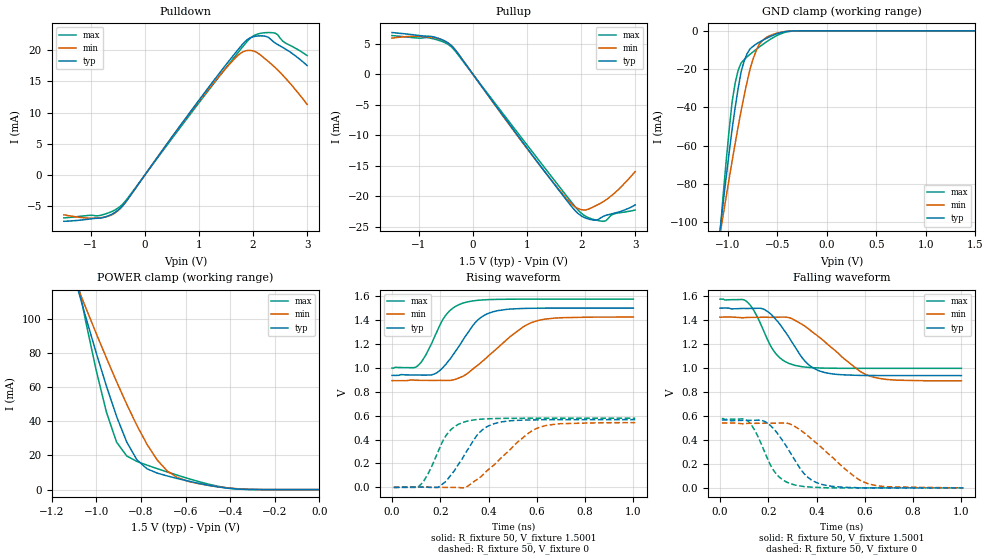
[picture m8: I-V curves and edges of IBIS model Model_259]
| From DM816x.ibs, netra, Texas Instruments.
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| Model based on original model for BSHTLTCSCDDVGPBFZ
|   Sub model FAST_5MA_5PER_P_1P5
[model]   Model_259
|[Description]  1.5V-3-STATE-X-FAST, 5MA, +-5%
|[Input Load]
|[Output Drive] FAST, 5MA
|Voltage   1.5V
|Mode   3-STATE
Model_type   3-state
Polarity   Non-Inverting
Enable   Active-Low
Cref =  15.0000pF
Rref =  100.0000M
Vref =  0V
Vmeas =  0.75005
C_comp   1.5249p   1.4275p   1.6205p
[Model Spec]
[Temperature Range]   25   125   -40
[Voltage Range]   1.5   1.425   1.575
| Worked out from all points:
|   slope of the pulldown table from 0 to 0.225 V, typ, clamps not added: 81.7 ohm
|   slope of the pullup table from 0 to 0.225 V, typ, clamps not added: 81.7 ohm
|   GND clamp passes 1 mA (typ) near -0.47 V on its own axis
|   POWER clamp passes 1 mA (typ) near -0.42 V on its own axis
|   rising waveform, R_fixture 50, V_fixture 1.5001: 20-80 % time 118ps typ, 187ps min, 89ps max; typ from 0.937 V to 1.5 V
|   rising waveform, R_fixture 50, V_fixture 0: 20-80 % time 112ps typ, 175ps min, 85.1ps max; typ from 0 V to 0.566 V
|   falling waveform, R_fixture 50, V_fixture 1.5001: 20-80 % time 117ps typ, 191ps min, 88.4ps max; typ from 1.5 V to 0.937 V
|   falling waveform, R_fixture 50, V_fixture 0: 20-80 % time 112ps typ, 184ps min, 84.9ps max; typ from 0.566 V to 0 V
[POWER_clamp]
-1.5V     321.7mA    260.6mA    415.9mA
-1.076V   114.2mA    115.8mA    116.9mA
-1.061V   107.2mA    110.9mA    107.1mA
-954.6mV  60.59mA    77.06mA    45.35mA
-909.2mV  42.85mA    63.21mA    27.81mA
-863.7mV  27.9mA     49.99mA    19.69mA
-818.2mV  17.49mA    37.63mA    16.52mA
-772.8mV  12.19mA    26.53mA    14.33mA
-681.9mV  7.985mA    10.89mA    10.33mA
-590.9mV  5.094mA    4.955mA    6.6mA
-363.7mV  298.5uA    465.2uA    297.6uA
0V        1.518nA    24.08nA    367.8pA
[Pulldown]
-1.5V     -7.45mA    -6.4mA     -6.9mA
-863.7mV  -6.95mA    -6.903mA   -6.565mA
-500mV    -5.682mA   -5.758mA   -5.339mA
-318.2mV  -3.897mA   -3.924mA   -3.728mA
1.046V    12.53mA    12.35mA    12.1mA
1.591V    18.69mA    18.02mA    18.2mA
1.818V    21.09mA    19.78mA    20.66mA
1.955V    22.02mA    19.97mA    21.99mA
2.091V    22.3mA     19.54mA    22.62mA
2.273V    22.11mA    18.26mA    22.84mA
2.364V    21.46mA    17.58mA    22.81mA
3V        17.55mA    11.32mA    19.14mA
[Pullup]
-1.5V     6.87mA     5.96mA     6.38mA
-818.2mV  6.271mA    6.141mA    6.005mA
-590.9mV  5.763mA    5.741mA    5.469mA
-409.1mV  4.8mA      4.791mA    4.587mA
1.227V    -14.81mA   -14.84mA   -14.21mA
1.727V    -20.63mA   -20.37mA   -19.92mA
1.909V    -22.57mA   -21.88mA   -21.95mA
2.046V    -23.45mA   -22.28mA   -23.09mA
2.227V    -23.93mA   -21.76mA   -23.82mA
2.409V    -23.32mA   -20.9mA    -24.13mA
2.591V    -22.85mA   -19.7mA    -22.97mA
3V        -21.43mA   -15.95mA   -22.28mA
[GND_clamp]
-1.5V     -310.1mA   -250.5mA   -402.5mA
-1.076V   -103.6mA   -106.2mA   -105.2mA
-1.046V   -89.81mA   -96.36mA   -86.02mA
-954.6mV  -51.22mA   -67.87mA   -36.88mA
-924.3mV  -40.08mA   -58.86mA   -27.29mA
-863.7mV  -21.24mA   -41.56mA   -16.73mA
-833.4mV  -15.8mA    -33.75mA   -15.03mA
-772.8mV  -9.345mA   -19.75mA   -12.19mA
-712.2mV  -6.928mA   -10.35mA   -9.704mA
-621.3mV  -4.261mA   -3.896mA   -6.225mA
-409.1mV  -337.1uA   -289.1uA   -618.9uA
1.5V      1.518nA    257.2nA    299pA
[Ramp]
dV/dt_f   0.45084/0.17883415n   0.425896/0.27079683n   0.4624/0.14098927n
dV/dt_r 0.45449408/0.17056745n 0.43634864/0.25170346n 0.46290125/0.13634761n
R_load = 50
[Rising Waveform]
R_fixture = 50
V_fixture = 1.5001
V_fixture_min = 1.425
V_fixture_max = 1.575
0s        937.3mV    893.3mV    997.8mV
105.5ps   940.3mV    896mV      1.015V
140.9ps   939.6mV    895.5mV    1.11V
190.7ps   965.5mV    895.3mV    1.322V
236.6ps   1.063V     894.9mV    1.472V
297.2ps   1.242V     932.8mV    1.544V
345.4ps   1.379V     1.007V     1.563V
389ps     1.446V     1.08V      1.57V
580.2ps   1.499V     1.38V      1.575V
1ns       1.5V       1.425V     1.575V
[Rising Waveform]
R_fixture = 50
V_fixture = 0
V_fixture_min = 0
V_fixture_max = 0
7.64ps    0V         0V         0V
113ps     3.206mV    2.933mV    11.95mV
147.8ps   2.243mV    2.369mV    106.8mV
189.5ps   0V         0V         291mV
238ps     87.51mV    0V         469.6mV
308.9ps   300.8mV    4.48mV     552.9mV
357.8ps   448.4mV    72.85mV    568.7mV
407.3ps   521mV      162.2mV    574.8mV
604.8ps   565.2mV    497.7mV    578.4mV
1.008ns   566.5mV    541.4mV    578.6mV
[Falling Waveform]
R_fixture = 50
V_fixture = 1.5001
V_fixture_min = 1.425
V_fixture_max = 1.575
0s        1.5V       1.424V     1.575V
110.7ps   1.496V     1.421V     1.554V
144.1ps   1.497V     1.422V     1.466V
184.6ps   1.487V     1.423V     1.293V
240.5ps   1.383V     1.424V     1.099V
310.6ps   1.177V     1.398V     1.022V
352.4ps   1.056V     1.348V     1.008V
403ps     982.7mV    1.27V      1.001V
612.2ps   937.4mV    938.9mV    997mV
1ns       936.6mV    892.7mV    997mV
[Falling Waveform]
R_fixture = 50
V_fixture = 0
V_fixture_min = 0
V_fixture_max = 0
7.64ps    565.9mV    540.6mV    577.7mV
117.8ps   562.8mV    538.2mV    552.8mV
155.7ps   564.9mV    538.7mV    434.1mV
201.9ps   533mV      539.3mV    220mV
243.8ps   438.5mV    540.8mV    92.95mV
291.6ps   292mV      531.3mV    34.75mV
349.5ps   116.5mV    457.9mV    10.7mV
395.4ps   47.6mV     380.2mV    4.436mV
607.7ps   0V         38.76mV    0V
1.008ns   0V         0V         0V
